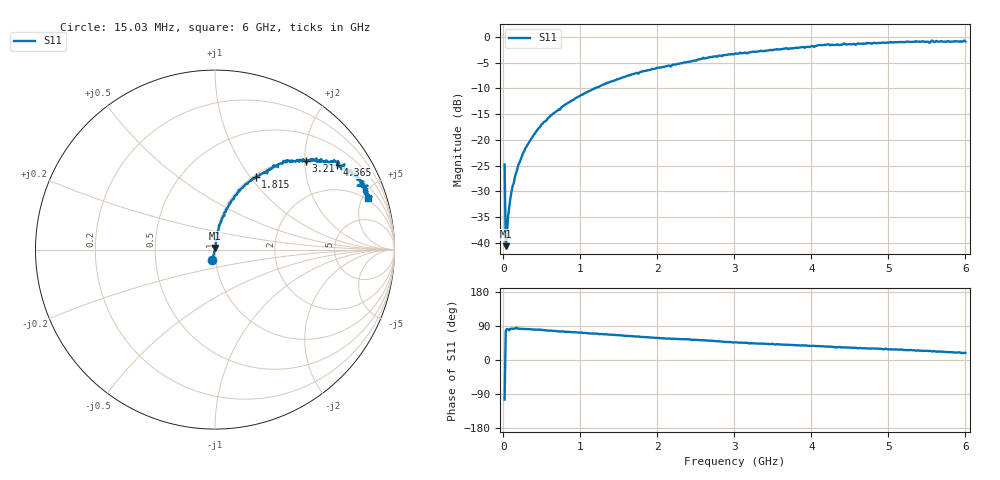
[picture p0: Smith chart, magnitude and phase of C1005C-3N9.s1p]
!	Network	Analyzer	HP8753E.07.74:	Oct	30	2002	Serial	No.	JP38451487
!	Hewlett-Packard
!	7	Sep	2009	8:23:06
!	Frequency	S11
#	HZ	S	RI	R	50
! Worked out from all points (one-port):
!   400 points, 15.03 MHz to 6 GHz, reference 50 ohm
!   lowest |S11| = -40.6 dB at 30.03 MHz (marker M1), VSWR 1.02, Z = 50.2 + j0.912 ohm
!   |S11| at or under -10 dB: start of sweep to 1.185 GHz
!   S11 on the Smith chart (normalised r, x): 15.03 MHz: 0.97, -0.11; 1.815 GHz: 1.03, +1.07; 3.21 GHz: 1.02, +2.03; 4.365 GHz: 0.96, +2.91; 6 GHz: 1.81, +5.51
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1.502992e7  -0.0144 -0.0558
3.002985e7  0.00203 0.00908
4.502978e7  0.00162 0.0117
6.00297e7  0.00282 0.0179
9.002955e7  0.0036 0.0269
1.200294e8  0.00452 0.0356
1.95029e8  0.00688 0.0574
2.850286e8  0.0117 0.0823
4.500278e8  0.0225 0.126
7.650262e8  0.0516 0.204
1.065025e9  0.0906 0.272
1.515022e9  0.166 0.357
1.815021e9  0.227 0.406
2.265019e9  0.309 0.451
3.015015e9  0.473 0.502
3.210014e9  0.508 0.495
3.765011e9  0.595 0.493
4.230009e9  0.692 0.482
4.365008e9  0.682 0.472
4.425008e9  0.722 0.475
4.515007e9  0.715 0.451
5.265004e9  0.806 0.391
5.445003e9  0.829 0.365
5.535002e9  0.795 0.357
5.565002e9  0.85 0.356
5.595002e9  0.815 0.354
5.625002e9  0.848 0.334
6e9  0.853 0.288
